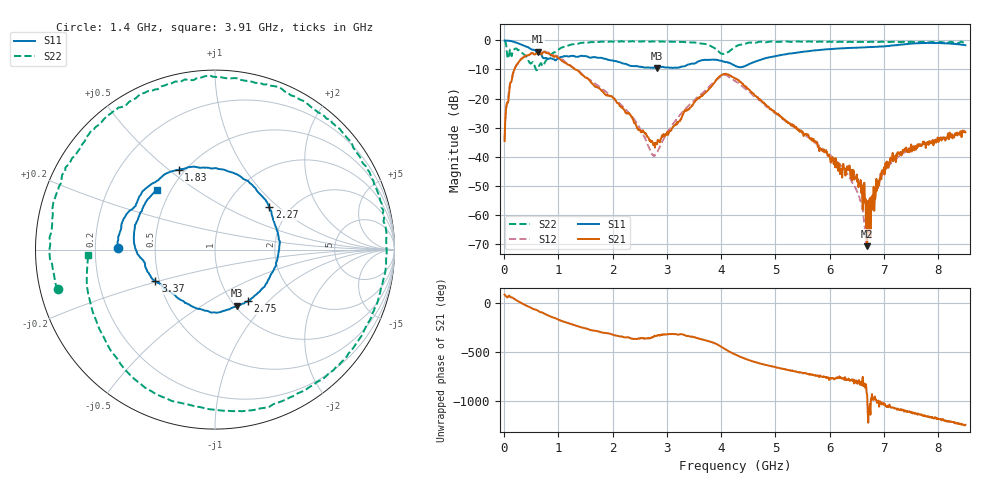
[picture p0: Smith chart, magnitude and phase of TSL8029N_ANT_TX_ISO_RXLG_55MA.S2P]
!Agilent Technologies,E5071C,MY46523237,B.13.01
!Date: Wed Oct 18 10:58:14 2023
!Data & Calibration Information:
!Freq	S11:SOLT2(ON)	S21:SOLT2(ON)	S12:SOLT2(ON)	S22:SOLT2(ON)
!PortZ  Port1:50+j0  Port2:50+j0
!Above PortZ is port z conversion or system Z0 setting when saving the data.
!When reading, reference impedance value at option line is always used.
# Hz S dB R 50
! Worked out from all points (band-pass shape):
!   850 points, 10 MHz to 8.5 GHz, reference 50 ohm
!   highest |S21| = -3.85 dB at 630 MHz (marker M1); lowest = -70.9 dB at 6.69 GHz (marker M2)
!   |S21| within 3 dB of the highest: 297 MHz to 1.055 GHz (758.4 MHz wide, 112 % of centre)
!   lowest |S11| = -9.5 dB at 2.81 GHz (marker M3), VSWR 2.01, Z = 50.9 - j35.9 ohm
!   |S11| at or under -10 dB: nowhere
!   |S22| runs from -10.3 to 0.0 dB; largest |S21 - S12| = 0.039
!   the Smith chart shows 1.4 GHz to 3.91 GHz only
!   S11 on the Smith chart (normalised r, x): 1.4 GHz: 0.30, +0.01; 1.83 GHz: 0.46, +0.54; 2.27 GHz: 1.57, +0.88; 2.75 GHz: 1.18, -0.77; 3.37 GHz: 0.48, -0.20; 3.91 GHz: 0.42, +0.36
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1e7  -0.01 -1.9  -34.64 85.6  -34.19 84.1  0.00 -9.4
3.7e8  -1.81 -67.7  -5.66 -15.6  -5.59 -15.4  -4.89 -151.5
6.3e8  -4.66 -104.5  -3.85 -81.7  -3.85 -80.0  -9.52 73.3
1.04e9  -5.74 -134.4  -6.55 -179.3  -6.08 -178.4  -2.65 -92.2
1.4e9  -5.37 179.3  -11.05 114.8  -10.92 117.5  -0.92 -165.7
1.43e9  -5.32 174.2  -11.76 110.0  -11.41 112.6  -0.84 -170.5
1.83e9  -6.22 114.5  -17.87 56.3  -16.99 56.0  -0.45 132.8
2.27e9  -8.30 38.3  -25.17 9.9  -24.41 2.9  -0.39 80.0
2.75e9  -9.33 -57.4  -36.03 11.0  -39.44 13.5  -0.37 24.5
2.81e9  -9.48 -69.0  -35.69 24.1  -38.90 39.5  -0.33 17.7
2.84e9  -9.42 -74.3  -34.31 33.8  -37.77 46.5  -0.39 14.3
3.37e9  -8.50 -152.0  -23.87 23.5  -22.97 25.5  -0.62 -52.4
3.7e9  -6.61 163.0  -18.20 -19.1  -17.43 -24.2  -1.20 -110.1
3.91e9  -6.69 134.2  -13.59 -57.5  -13.62 -66.8  -3.01 -177.7
4.07e9  -7.40 114.0  -11.54 -109.0  -11.94 -116.1  -4.56 80.7
4.26e9  -8.77 93.9  -13.15 -165.2  -14.06 -169.5  -2.22 -20.1
4.72e9  -6.68 56.4  -20.40 103.7  -20.80 104.7  -0.41 -107.4
5.67e9  -3.54 -75.7  -33.69 -9.5  -34.37 -8.5  -0.45 163.6
6.69e9  -2.31 -178.0  -70.86 143.2  -69.26 131.2  -0.52 78.1
7.09e9  -1.91 144.9  -42.55 27.7  -43.24 26.6  -0.53 43.1
7.76e9  -0.88 72.7  -35.33 -67.3  -35.49 -69.4  -0.65 -16.1
8.5e9  -1.64 -18.8  -31.62 -161.8  -30.90 -165.3  -1.04 -89.7
